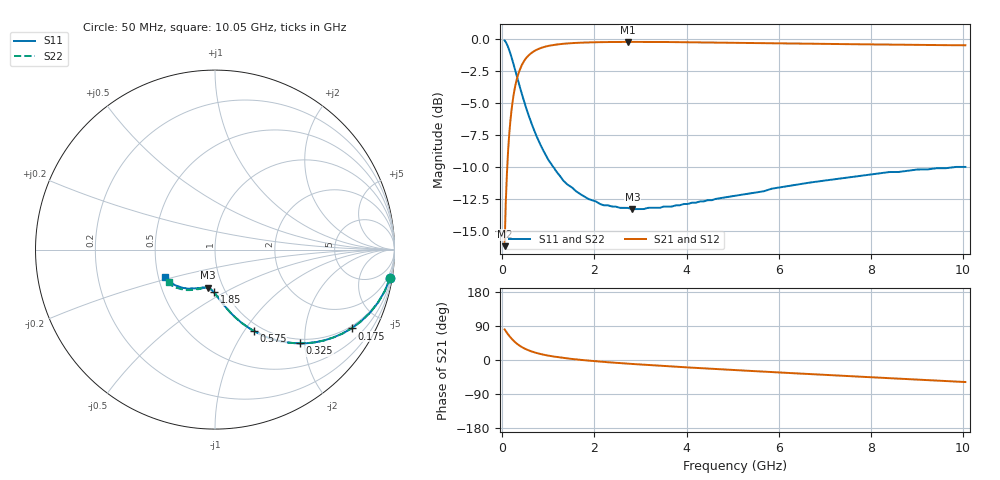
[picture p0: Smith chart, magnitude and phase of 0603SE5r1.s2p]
! AVX Thin Film Operation		Date: August 2001
! Description: Accu-P® Series, Thin Film, SMD, RF Capacitor
! Part Number: 06035J5R1ABT
! 50 MHz  -  10.05 GHz
! Serial Measurements
# mhz S db R 50
!	S11		S21		S12		S22
!	dB	Phase	dB	Phase	dB	Phase	dB	Phase
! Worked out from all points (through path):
!   401 points, 50 MHz to 10.05 GHz, reference 50 ohm
!   highest |S21| = -0.22 dB at 2.725 GHz (marker M1); lowest = -16.2 dB at 50 MHz (marker M2)
!   group delay of S21, straight-line fit = 23.7 ps
!   lowest |S11| = -13.3 dB at 2.825 GHz (marker M3), VSWR 1.55, Z = 42.2 - j18.8 ohm
!   |S11| at or under -10 dB: 1.105 GHz to 9.875 GHz (8.77 GHz wide, 160 % of centre); 9.925 GHz to end of sweep
!   |S22| runs from -13.3 to -0.1 dB; largest |S21 - S12| = 0
!   S11 on the Smith chart (normalised r, x): 50 MHz: 1, -12; 175 MHz: 0.91, -3.51; 325 MHz: 0.91, -1.90; 575 MHz: 0.91, -1.10; 1.85 GHz: 0.88, -0.45; 10.05 GHz: 0.54, -0.19
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50  -0.10 -9.3  -16.20 80.7  -16.20 80.7  -0.10 -9.3
75  -0.23 -13.8  -12.81 76.2  -12.81 76.2  -0.23 -13.8
125  -0.62 -22.3  -8.78 67.6  -8.78 67.6  -0.62 -22.3
175  -1.13 -30.0  -6.42 60.0  -6.42 60.0  -1.13 -30.0
250  -2.04 -39.8  -4.26 50.2  -4.26 50.2  -2.04 -39.8
325  -3.02 -47.7  -3.00 42.3  -3.00 42.3  -3.02 -47.7
375  -3.67 -52.1  -2.44 37.9  -2.44 37.9  -3.67 -52.1
450  -4.60 -57.7  -1.85 32.3  -1.85 32.3  -4.60 -57.7
575  -6.00 -64.6  -1.26 25.3  -1.26 25.3  -6.00 -64.6
750  -7.65 -71.6  -0.82 18.3  -0.82 18.3  -7.65 -71.6
975  -9.27 -77.8  -0.55 12.1  -0.55 12.1  -9.27 -77.8
1350  -11.17 -85.0  -0.35 5.0  -0.35 5.0  -11.09 -84.8
1725  -12.20 -90.0  -0.28 0.0  -0.28 0.0  -12.20 -89.7
1850  -12.48 -91.4  -0.26 -1.4  -0.26 -1.4  -12.48 -91.0
2175  -12.97 -94.8  -0.23 -4.8  -0.23 -4.8  -12.90 -94.3
2725  -13.21 -100.0  -0.22 -9.7  -0.22 -9.7  -13.20 -99.0
2825  -13.30 -101.0  -0.22 -10.5  -0.22 -10.5  -13.22 -99.8
3400  -13.20 -105.8  -0.22 -15.0  -0.22 -15.0  -13.20 -104.0
5050  -12.26 -117.4  -0.28 -26.6  -0.28 -26.6  -12.26 -115.4
6725  -11.20 -129.0  -0.36 -37.4  -0.36 -37.4  -11.20 -125.0
8400  -10.40 -140.1  -0.43 -48.0  -0.43 -48.0  -10.39 -135.1
10050  -10.00 -150.8  -0.48 -58.1  -0.48 -58.1  -9.98 -144.8
